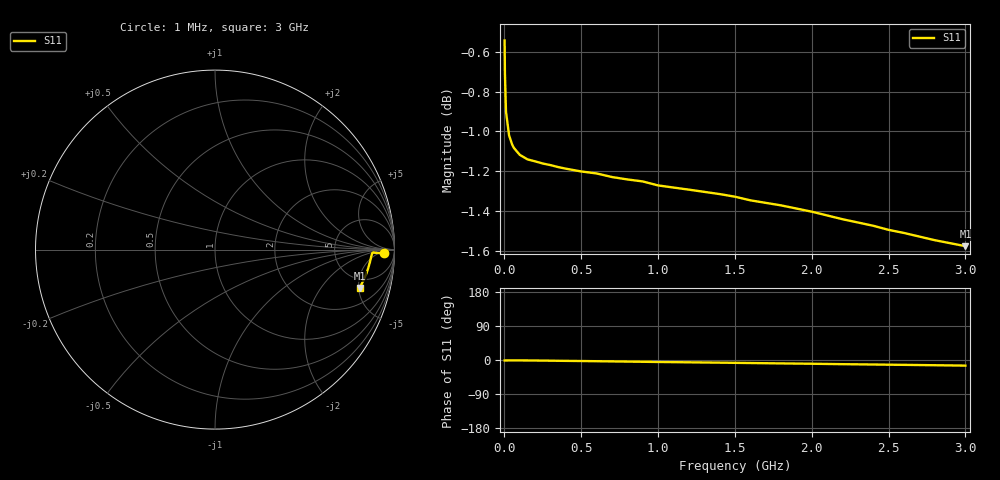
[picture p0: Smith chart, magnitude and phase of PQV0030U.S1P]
! SIEMENS Small Signal Semiconductors
! BAR64-04
! Si PIN Diode in SOT23 (2 diodes in series, pin 3 open)
! IF = 0.03 mA
! S-Parameters:  July  1992
# GHz  S  MA  R  50
!  f  S11
! GHz  MAG  ANG
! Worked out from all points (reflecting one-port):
!   33 points, 1 MHz to 3 GHz, reference 50 ohm
!   lowest |S11| = -1.6 dB at 3 GHz (marker M1), VSWR 11.06, Z = 184 - j257 ohm
!   phase of S11 starts at -1 deg and turns -14 deg over the sweep
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0.001  0.9394 -1.2
0.003  0.9221 -1.2
0.01  0.9015 -1.2
0.03  0.8893 -1.1
0.05  0.8846 -1.0
0.06  0.883 -1.0
0.08  0.8811 -1.1
0.1  0.8793 -1.1
0.15  0.877 -1.2
0.3  0.8741 -1.8
0.35  0.8731 -2.1
0.4  0.8723 -2.3
0.5  0.8709 -2.7
0.6  0.8699 -3.2
0.8  0.8669 -4.2
0.9  0.8659 -4.7
1  0.8639 -5.2
1.2  0.8618 -6.1
1.4  0.8596 -7.0
1.6  0.8565 -8.0
1.8  0.854 -9.0
2  0.8509 -9.9
2.2  0.8472 -11.0
2.4  0.844 -11.9
2.5  0.842 -12.4
2.6  0.8405 -12.8
2.8  0.837 -13.8
3  0.8341 -14.8
